(* Logix 5000 AddOnInstructionDefinition export Banner_EZAK2_PD_v4; software revision 33.00 *)

TYPE Banner_EZAK2_PDI_0_v4 :   // Process Data 0 - Array Measurement
STRUCT
   Active_Measure_1 : DINT;
   Active_Measure_2 : DINT;
END_STRUCT
END_TYPE

TYPE Banner_EZAK2_PDI_128_v4 :   // Process Data 128 - Channel State 1 "OR"
STRUCT
   Beams : INT[15];
END_STRUCT
END_TYPE

TYPE Banner_EZAK2_PDI_129_v4 :   // Process Data 129 - Channel State 2 "AND"
STRUCT
   Beams : INT[15];
END_STRUCT
END_TYPE

TYPE Banner_EZAK2_PDI_1_v4 :   // Process Data 1 - Straight Scan Measurements
STRUCT
   FBB : DINT;   // First Beam Blocked
   LBB : DINT;   // Last Beam Blocked
   TBB : DINT;   // Total Beams Blocked
   Transitions : DINT;
   CBB : DINT;   // Contiguous Beams Blocked
   FBM : DINT;   // First Beam Made
   LBM : DINT;   // Last Beam Made
   TBM : DINT;   // Total Beam Made
   CBM : DINT;   // Contiguous Beams Made
   MBB : DINT;   // Middle Beam Blocked
   CFBB : DINT;   // Contiguous First Beam Blocked
   CLBB : DINT;   // Contiguous Last Beam Blocked
END_STRUCT
END_TYPE

TYPE Banner_EZAK2_PDI_2_v4 :   // Process Data 2 - Edge Scan Measurement
STRUCT
   FBB : DINT;   // First Beam Blocked
   LBB : DINT;   // Last Beam Blocked
   TBB : DINT;   // Total Beams Blocked
   CBB : DINT;   // Contiguous Beam Blocked
   MBB : DINT;   // Middle Beam Blocked
   OD : DINT;   // Outer Diameter
   ID : DINT;   // Inner Diameter
   CFBB : DINT;   // Contiguous First Beam Blocked
   CLBB : DINT;   // Contiguous Last Beam Blocked
   Object_1_FBB : DINT;   // Object 1 First Beam Blocked
   Object_1_LBB : DINT;   // Object 1 Last Beam Blocked
   Object_2_FBB : DINT;   // Object 2 First Beam Blocked
   Object_2_LBB : DINT;   // Object 2 Last Beam Blocked
   Object_3_FBB : DINT;   // Object 3 First Beam Blocked
   Object_3_LBB : DINT;   // Object 3 Last Beam Blocked
END_STRUCT
END_TYPE

TYPE Banner_EZAK2_PDI_v4 :   // UDT that records the converted prcoess data.
STRUCT
   Array_Measure : Banner_EZAK2_PDI_0_v4;
   Straight_Scan : Banner_EZAK2_PDI_1_v4;
   Edge_Scan : Banner_EZAK2_PDI_2_v4;
   CS_1 : Banner_EZAK2_PDI_128_v4;   // Channel State 1: OR Beam States for Sticks longer than
   CS_2 : Banner_EZAK2_PDI_129_v4;   // Channel State 2: AND Beam States for Sticks longer than
   Data_In : SINT[30];
END_STRUCT
END_TYPE

ADD_ON_INSTRUCTION Banner_EZAK2_PD_v4   (* revision 4.0, vendor Banner Engineering *)
// Takes the raw SINT information and converts that data into actual information. Used with EZ-Array K2.
VAR_IN_OUT
   Process_Data : Banner_EZAK2_PDI_v4; {required}
END_VAR
VAR_INPUT
   UserProcess : INT; {required}
   Byte_Swap : BOOL; {required}
END_VAR
VAR
   Temp_Measure : DINT[15]; {access None}
   Temp_Byte : SINT[30]; {access None}
   Index1 : DINT; {access None}
   Update : BOOL; {access None}
   Index2 : DINT; {access None}
   Temp : DINT[15]; {access None}
END_VAR

ROUTINE Logic   (* ladder *)
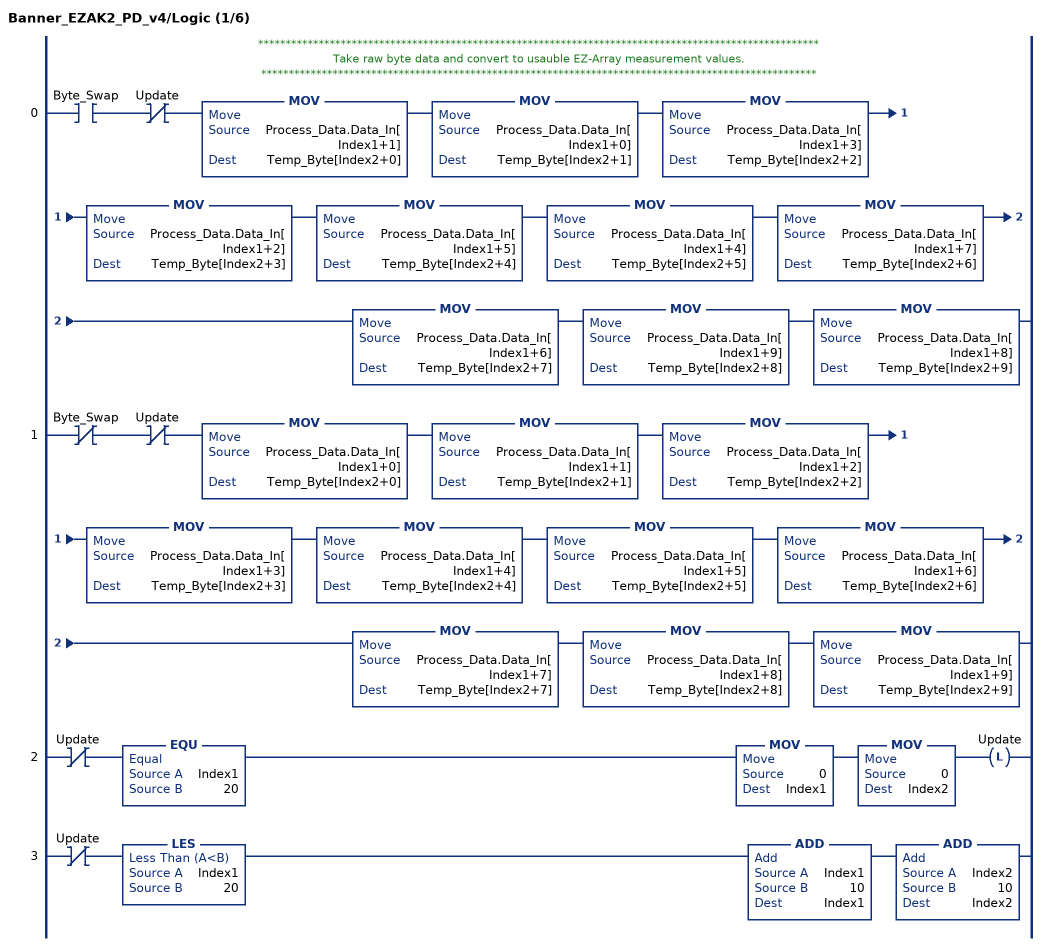
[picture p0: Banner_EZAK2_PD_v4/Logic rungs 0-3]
   // ******************************************************************************************************
   // Take raw byte data and convert to usauble EZ-Array measurement values.
   // *****************************************************************************************************
   0: XIC(Byte_Swap)XIO(Update)MOV(Process_Data.Data_In[Index1+1],Temp_Byte[Index2+0])MOV(Process_Data.Data_In[Index1+0],Temp_Byte[Index2+1])MOV(Process_Data.Data_In[Index1+3],Temp_Byte[Index2+2])MOV(Process_Data.Data_In[Index1+2],Temp_Byte[Index2+3])MOV(Process_Data.Data_In[Index1+5],Temp_Byte[Index2+4])MOV(Process_Data.Data_In[Index1+4],Temp_Byte[Index2+5])MOV(Process_Data.Data_In[Index1+7],Temp_Byte[Index2+6])MOV(Process_Data.Data_In[Index1+6],Temp_Byte[Index2+7])MOV(Process_Data.Data_In[Index1+9],Temp_Byte[Index2+8])MOV(Process_Data.Data_In[Index1+8],Temp_Byte[Index2+9]);
   1: XIO(Byte_Swap)XIO(Update)MOV(Process_Data.Data_In[Index1+0],Temp_Byte[Index2+0])MOV(Process_Data.Data_In[Index1+1],Temp_Byte[Index2+1])MOV(Process_Data.Data_In[Index1+2],Temp_Byte[Index2+2])MOV(Process_Data.Data_In[Index1+3],Temp_Byte[Index2+3])MOV(Process_Data.Data_In[Index1+4],Temp_Byte[Index2+4])MOV(Process_Data.Data_In[Index1+5],Temp_Byte[Index2+5])MOV(Process_Data.Data_In[Index1+6],Temp_Byte[Index2+6])MOV(Process_Data.Data_In[Index1+7],Temp_Byte[Index2+7])MOV(Process_Data.Data_In[Index1+8],Temp_Byte[Index2+8])MOV(Process_Data.Data_In[Index1+9],Temp_Byte[Index2+9]);
   2: XIO(Update)EQU(Index1,20)MOV(0,Index1)MOV(0,Index2)OTL(Update);
   3: XIO(Update)LES(Index1,20)ADD(Index1,10,Index1)ADD(Index2,10,Index2);
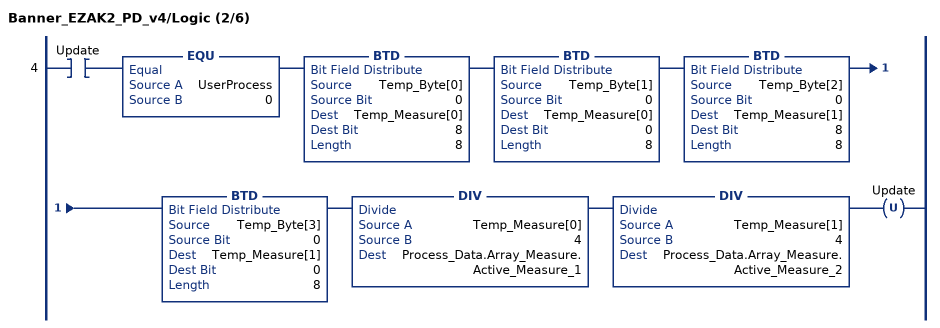
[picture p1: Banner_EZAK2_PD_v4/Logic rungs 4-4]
   4: XIC(Update)EQU(UserProcess,0)BTD(Temp_Byte[0],0,Temp_Measure[0],8,8)BTD(Temp_Byte[1],0,Temp_Measure[0],0,8)BTD(Temp_Byte[2],0,Temp_Measure[1],8,8)BTD(Temp_Byte[3],0,Temp_Measure[1],0,8)DIV(Temp_Measure[0],4,Process_Data.Array_Measure.Active_Measure_1)DIV(Temp_Measure[1],4,Process_Data.Array_Measure.Active_Measure_2)OTU(Update);
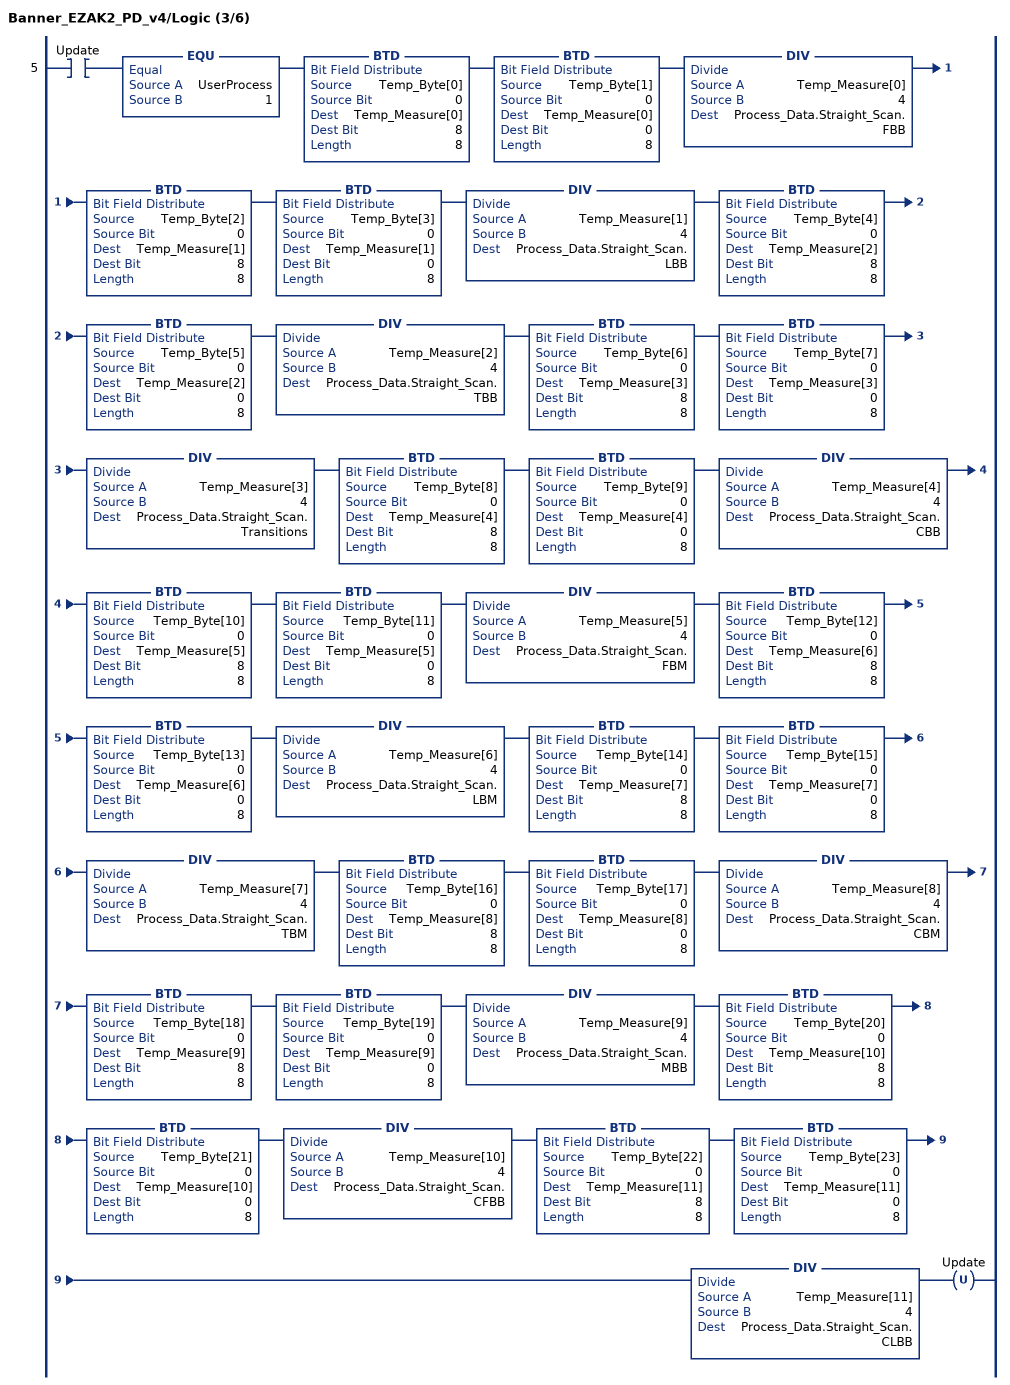
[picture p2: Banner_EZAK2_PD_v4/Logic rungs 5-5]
   5: XIC(Update)EQU(UserProcess,1)BTD(Temp_Byte[0],0,Temp_Measure[0],8,8)BTD(Temp_Byte[1],0,Temp_Measure[0],0,8)DIV(Temp_Measure[0],4,Process_Data.Straight_Scan.FBB)BTD(Temp_Byte[2],0,Temp_Measure[1],8,8)BTD(Temp_Byte[3],0,Temp_Measure[1],0,8)DIV(Temp_Measure[1],4,Process_Data.Straight_Scan.LBB)BTD(Temp_Byte[4],0,Temp_Measure[2],8,8)BTD(Temp_Byte[5],0,Temp_Measure[2],0,8)DIV(Temp_Measure[2],4,Process_Data.Straight_Scan.TBB)BTD(Temp_Byte[6],0,Temp_Measure[3],8,8)BTD(Temp_Byte[7],0,Temp_Measure[3],0,8)DIV(Temp_Measure[3],4,Process_Data.Straight_Scan.Transitions)BTD(Temp_Byte[8],0,Temp_Measure[4],8,8)BTD(Temp_Byte[9],0,Temp_Measure[4],0,8)DIV(Temp_Measure[4],4,Process_Data.Straight_Scan.CBB)BTD(Temp_Byte[10],0,Temp_Measure[5],8,8)BTD(Temp_Byte[11],0,Temp_Measure[5],0,8)DIV(Temp_Measure[5],4,Process_Data.Straight_Scan.FBM)BTD(Temp_Byte[12],0,Temp_Measure[6],8,8)BTD(Temp_Byte[13],0,Temp_Measure[6],0,8)DIV(Temp_Measure[6],4,Process_Data.Straight_Scan.LBM)BTD(Temp_Byte[14],0,Temp_Measure[7],8,8)BTD(Temp_Byte[15],0,Temp_Measure[7],0,8)DIV(Temp_Measure[7],4,Process_Data.Straight_Scan.TBM)BTD(Temp_Byte[16],0,Temp_Measure[8],8,8)BTD(Temp_Byte[17],0,Temp_Measure[8],0,8)DIV(Temp_Measure[8],4,Process_Data.Straight_Scan.CBM)BTD(Temp_Byte[18],0,Temp_Measure[9],8,8)BTD(Temp_Byte[19],0,Temp_Measure[9],0,8)DIV(Temp_Measure[9],4,Process_Data.Straight_Scan.MBB)BTD(Temp_Byte[20],0,Temp_Measure[10],8,8)BTD(Temp_Byte[21],0,Temp_Measure[10],0,8)DIV(Temp_Measure[10],4,Process_Data.Straight_Scan.CFBB)BTD(Temp_Byte[22],0,Temp_Measure[11],8,8)BTD(Temp_Byte[23],0,Temp_Measure[11],0,8)DIV(Temp_Measure[11],4,Process_Data.Straight_Scan.CLBB)OTU(Update);
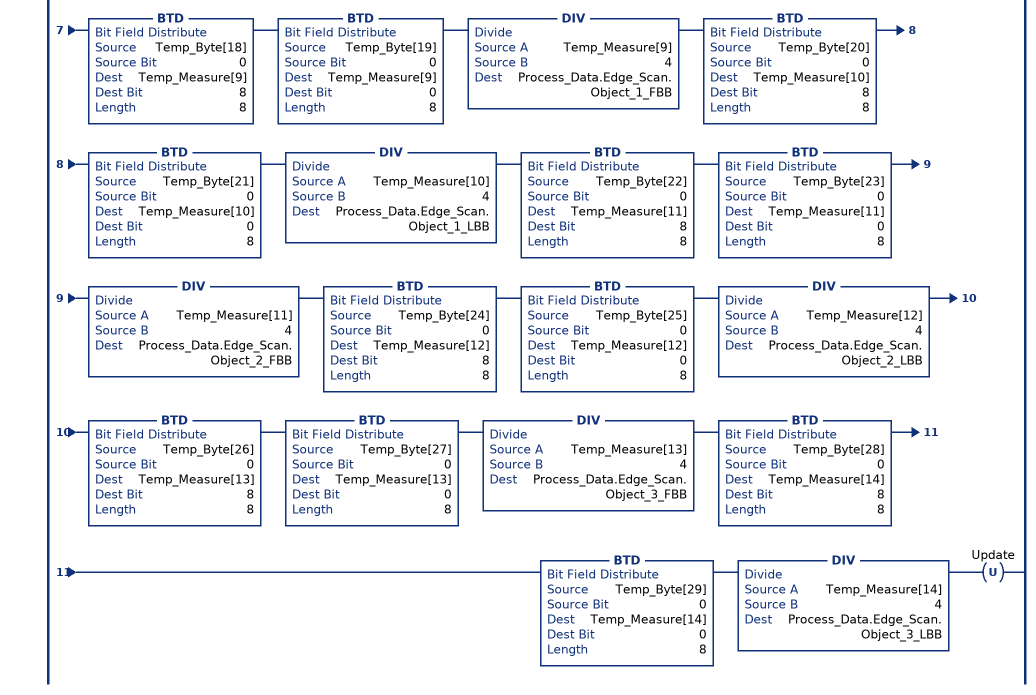
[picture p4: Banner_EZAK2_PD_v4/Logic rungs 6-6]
   6: XIC(Update)EQU(UserProcess,2)BTD(Temp_Byte[0],0,Temp_Measure[0],8,8)BTD(Temp_Byte[1],0,Temp_Measure[0],0,8)DIV(Temp_Measure[0],4,Process_Data.Edge_Scan.FBB)BTD(Temp_Byte[2],0,Temp_Measure[1],8,8)BTD(Temp_Byte[3],0,Temp_Measure[1],0,8)DIV(Temp_Measure[1],4,Process_Data.Edge_Scan.LBB)BTD(Temp_Byte[4],0,Temp_Measure[2],8,8)BTD(Temp_Byte[5],0,Temp_Measure[2],0,8)DIV(Temp_Measure[2],4,Process_Data.Edge_Scan.TBB)BTD(Temp_Byte[6],0,Temp_Measure[3],8,8)BTD(Temp_Byte[7],0,Temp_Measure[3],0,8)DIV(Temp_Measure[3],4,Process_Data.Edge_Scan.CBB)BTD(Temp_Byte[8],0,Temp_Measure[4],8,8)BTD(Temp_Byte[9],0,Temp_Measure[4],0,8)DIV(Temp_Measure[4],4,Process_Data.Edge_Scan.MBB)BTD(Temp_Byte[10],0,Temp_Measure[5],8,8)BTD(Temp_Byte[11],0,Temp_Measure[5],0,8)DIV(Temp_Measure[5],4,Process_Data.Edge_Scan.OD)BTD(Temp_Byte[12],0,Temp_Measure[6],8,8)BTD(Temp_Byte[13],0,Temp_Measure[6],0,8)DIV(Temp_Measure[6],4,Process_Data.Edge_Scan.ID)BTD(Temp_Byte[14],0,Temp_Measure[7],8,8)BTD(Temp_Byte[15],0,Temp_Measure[7],0,8)DIV(Temp_Measure[7],4,Process_Data.Edge_Scan.CFBB)BTD(Temp_Byte[16],0,Temp_Measure[8],8,8)BTD(Temp_Byte[17],0,Temp_Measure[8],0,8)DIV(Temp_Measure[8],4,Process_Data.Edge_Scan.CLBB)BTD(Temp_Byte[18],0,Temp_Measure[9],8,8)BTD(Temp_Byte[19],0,Temp_Measure[9],0,8)DIV(Temp_Measure[9],4,Process_Data.Edge_Scan.Object_1_FBB)BTD(Temp_Byte[20],0,Temp_Measure[10],8,8)BTD(Temp_Byte[21],0,Temp_Measure[10],0,8)DIV(Temp_Measure[10],4,Process_Data.Edge_Scan.Object_1_LBB)BTD(Temp_Byte[22],0,Temp_Measure[11],8,8)BTD(Temp_Byte[23],0,Temp_Measure[11],0,8)DIV(Temp_Measure[11],4,Process_Data.Edge_Scan.Object_2_FBB)BTD(Temp_Byte[24],0,Temp_Measure[12],8,8)BTD(Temp_Byte[25],0,Temp_Measure[12],0,8)DIV(Temp_Measure[12],4,Process_Data.Edge_Scan.Object_2_LBB)BTD(Temp_Byte[26],0,Temp_Measure[13],8,8)BTD(Temp_Byte[27],0,Temp_Measure[13],0,8)DIV(Temp_Measure[13],4,Process_Data.Edge_Scan.Object_3_FBB)BTD(Temp_Byte[28],0,Temp_Measure[14],8,8)BTD(Temp_Byte[29],0,Temp_Measure[14],0,8)DIV(Temp_Measure[14],4,Process_Data.Edge_Scan.Object_3_LBB)OTU(Update);
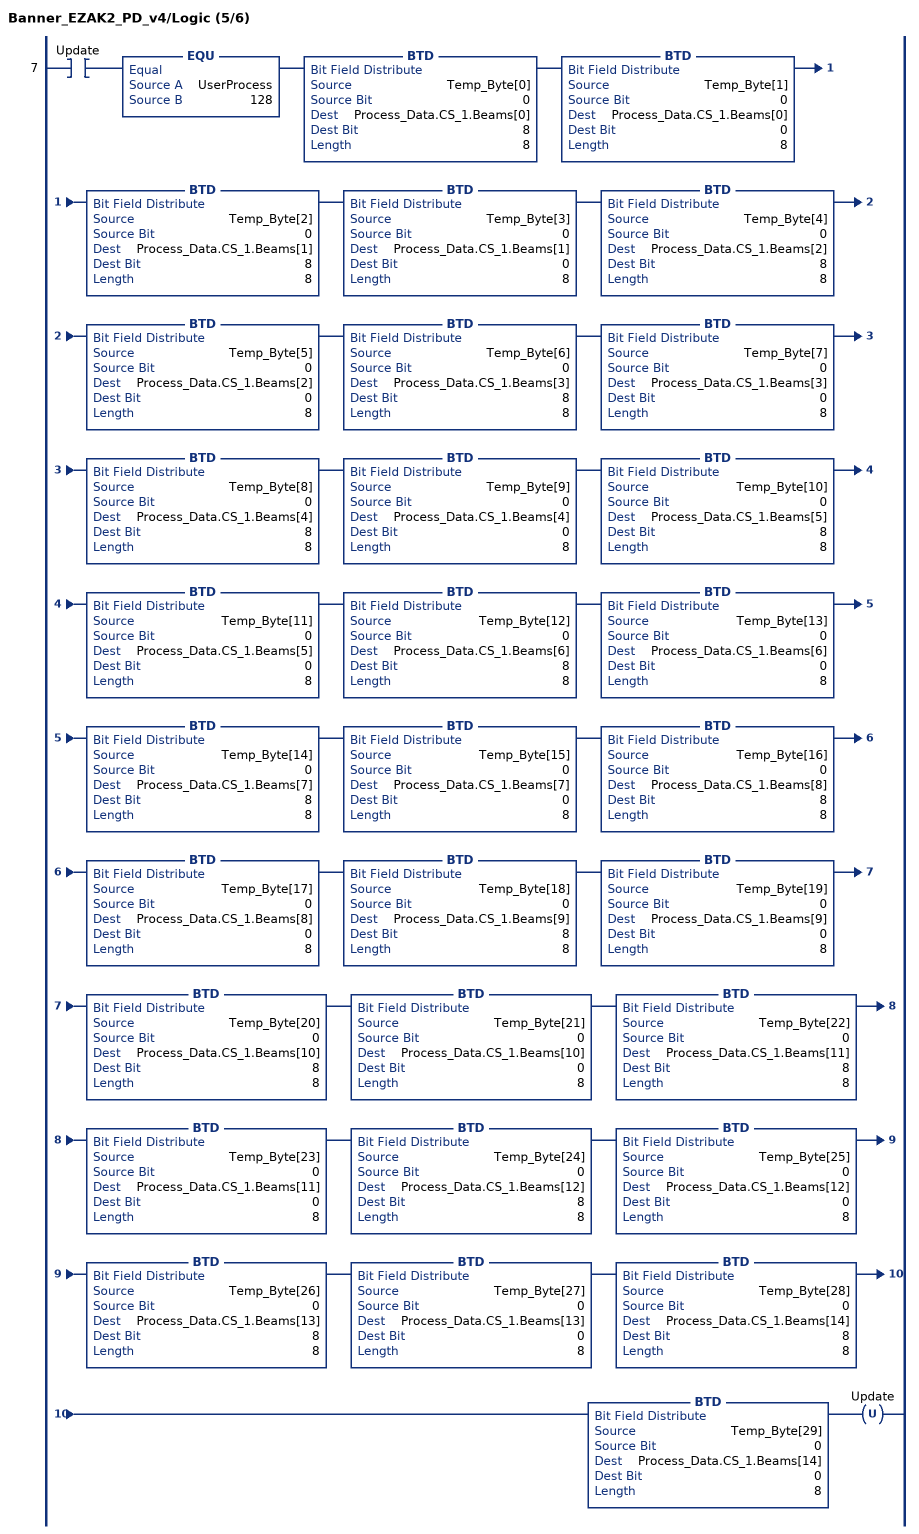
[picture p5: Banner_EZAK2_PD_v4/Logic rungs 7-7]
   7: XIC(Update)EQU(UserProcess,128)BTD(Temp_Byte[0],0,Process_Data.CS_1.Beams[0],8,8)BTD(Temp_Byte[1],0,Process_Data.CS_1.Beams[0],0,8)BTD(Temp_Byte[2],0,Process_Data.CS_1.Beams[1],8,8)BTD(Temp_Byte[3],0,Process_Data.CS_1.Beams[1],0,8)BTD(Temp_Byte[4],0,Process_Data.CS_1.Beams[2],8,8)BTD(Temp_Byte[5],0,Process_Data.CS_1.Beams[2],0,8)BTD(Temp_Byte[6],0,Process_Data.CS_1.Beams[3],8,8)BTD(Temp_Byte[7],0,Process_Data.CS_1.Beams[3],0,8)BTD(Temp_Byte[8],0,Process_Data.CS_1.Beams[4],8,8)BTD(Temp_Byte[9],0,Process_Data.CS_1.Beams[4],0,8)BTD(Temp_Byte[10],0,Process_Data.CS_1.Beams[5],8,8)BTD(Temp_Byte[11],0,Process_Data.CS_1.Beams[5],0,8)BTD(Temp_Byte[12],0,Process_Data.CS_1.Beams[6],8,8)BTD(Temp_Byte[13],0,Process_Data.CS_1.Beams[6],0,8)BTD(Temp_Byte[14],0,Process_Data.CS_1.Beams[7],8,8)BTD(Temp_Byte[15],0,Process_Data.CS_1.Beams[7],0,8)BTD(Temp_Byte[16],0,Process_Data.CS_1.Beams[8],8,8)BTD(Temp_Byte[17],0,Process_Data.CS_1.Beams[8],0,8)BTD(Temp_Byte[18],0,Process_Data.CS_1.Beams[9],8,8)BTD(Temp_Byte[19],0,Process_Data.CS_1.Beams[9],0,8)BTD(Temp_Byte[20],0,Process_Data.CS_1.Beams[10],8,8)BTD(Temp_Byte[21],0,Process_Data.CS_1.Beams[10],0,8)BTD(Temp_Byte[22],0,Process_Data.CS_1.Beams[11],8,8)BTD(Temp_Byte[23],0,Process_Data.CS_1.Beams[11],0,8)BTD(Temp_Byte[24],0,Process_Data.CS_1.Beams[12],8,8)BTD(Temp_Byte[25],0,Process_Data.CS_1.Beams[12],0,8)BTD(Temp_Byte[26],0,Process_Data.CS_1.Beams[13],8,8)BTD(Temp_Byte[27],0,Process_Data.CS_1.Beams[13],0,8)BTD(Temp_Byte[28],0,Process_Data.CS_1.Beams[14],8,8)BTD(Temp_Byte[29],0,Process_Data.CS_1.Beams[14],0,8)OTU(Update);
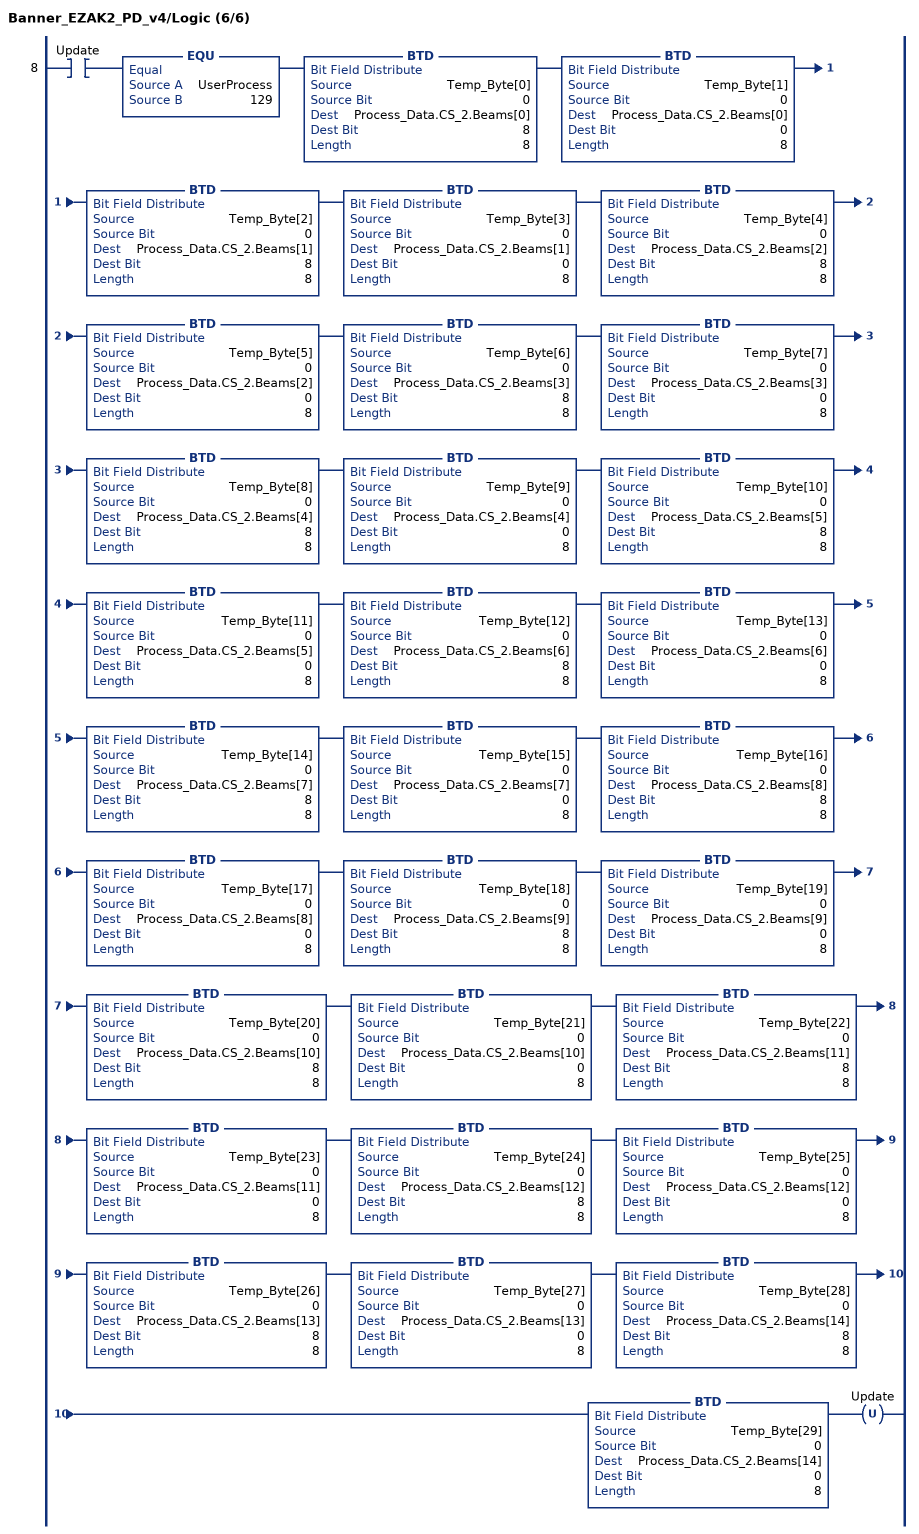
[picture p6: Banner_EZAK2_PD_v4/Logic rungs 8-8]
   8: XIC(Update)EQU(UserProcess,129)BTD(Temp_Byte[0],0,Process_Data.CS_2.Beams[0],8,8)BTD(Temp_Byte[1],0,Process_Data.CS_2.Beams[0],0,8)BTD(Temp_Byte[2],0,Process_Data.CS_2.Beams[1],8,8)BTD(Temp_Byte[3],0,Process_Data.CS_2.Beams[1],0,8)BTD(Temp_Byte[4],0,Process_Data.CS_2.Beams[2],8,8)BTD(Temp_Byte[5],0,Process_Data.CS_2.Beams[2],0,8)BTD(Temp_Byte[6],0,Process_Data.CS_2.Beams[3],8,8)BTD(Temp_Byte[7],0,Process_Data.CS_2.Beams[3],0,8)BTD(Temp_Byte[8],0,Process_Data.CS_2.Beams[4],8,8)BTD(Temp_Byte[9],0,Process_Data.CS_2.Beams[4],0,8)BTD(Temp_Byte[10],0,Process_Data.CS_2.Beams[5],8,8)BTD(Temp_Byte[11],0,Process_Data.CS_2.Beams[5],0,8)BTD(Temp_Byte[12],0,Process_Data.CS_2.Beams[6],8,8)BTD(Temp_Byte[13],0,Process_Data.CS_2.Beams[6],0,8)BTD(Temp_Byte[14],0,Process_Data.CS_2.Beams[7],8,8)BTD(Temp_Byte[15],0,Process_Data.CS_2.Beams[7],0,8)BTD(Temp_Byte[16],0,Process_Data.CS_2.Beams[8],8,8)BTD(Temp_Byte[17],0,Process_Data.CS_2.Beams[8],0,8)BTD(Temp_Byte[18],0,Process_Data.CS_2.Beams[9],8,8)BTD(Temp_Byte[19],0,Process_Data.CS_2.Beams[9],0,8)BTD(Temp_Byte[20],0,Process_Data.CS_2.Beams[10],8,8)BTD(Temp_Byte[21],0,Process_Data.CS_2.Beams[10],0,8)BTD(Temp_Byte[22],0,Process_Data.CS_2.Beams[11],8,8)BTD(Temp_Byte[23],0,Process_Data.CS_2.Beams[11],0,8)BTD(Temp_Byte[24],0,Process_Data.CS_2.Beams[12],8,8)BTD(Temp_Byte[25],0,Process_Data.CS_2.Beams[12],0,8)BTD(Temp_Byte[26],0,Process_Data.CS_2.Beams[13],8,8)BTD(Temp_Byte[27],0,Process_Data.CS_2.Beams[13],0,8)BTD(Temp_Byte[28],0,Process_Data.CS_2.Beams[14],8,8)BTD(Temp_Byte[29],0,Process_Data.CS_2.Beams[14],0,8)OTU(Update);
END_ROUTINE
END_ADD_ON_INSTRUCTION
